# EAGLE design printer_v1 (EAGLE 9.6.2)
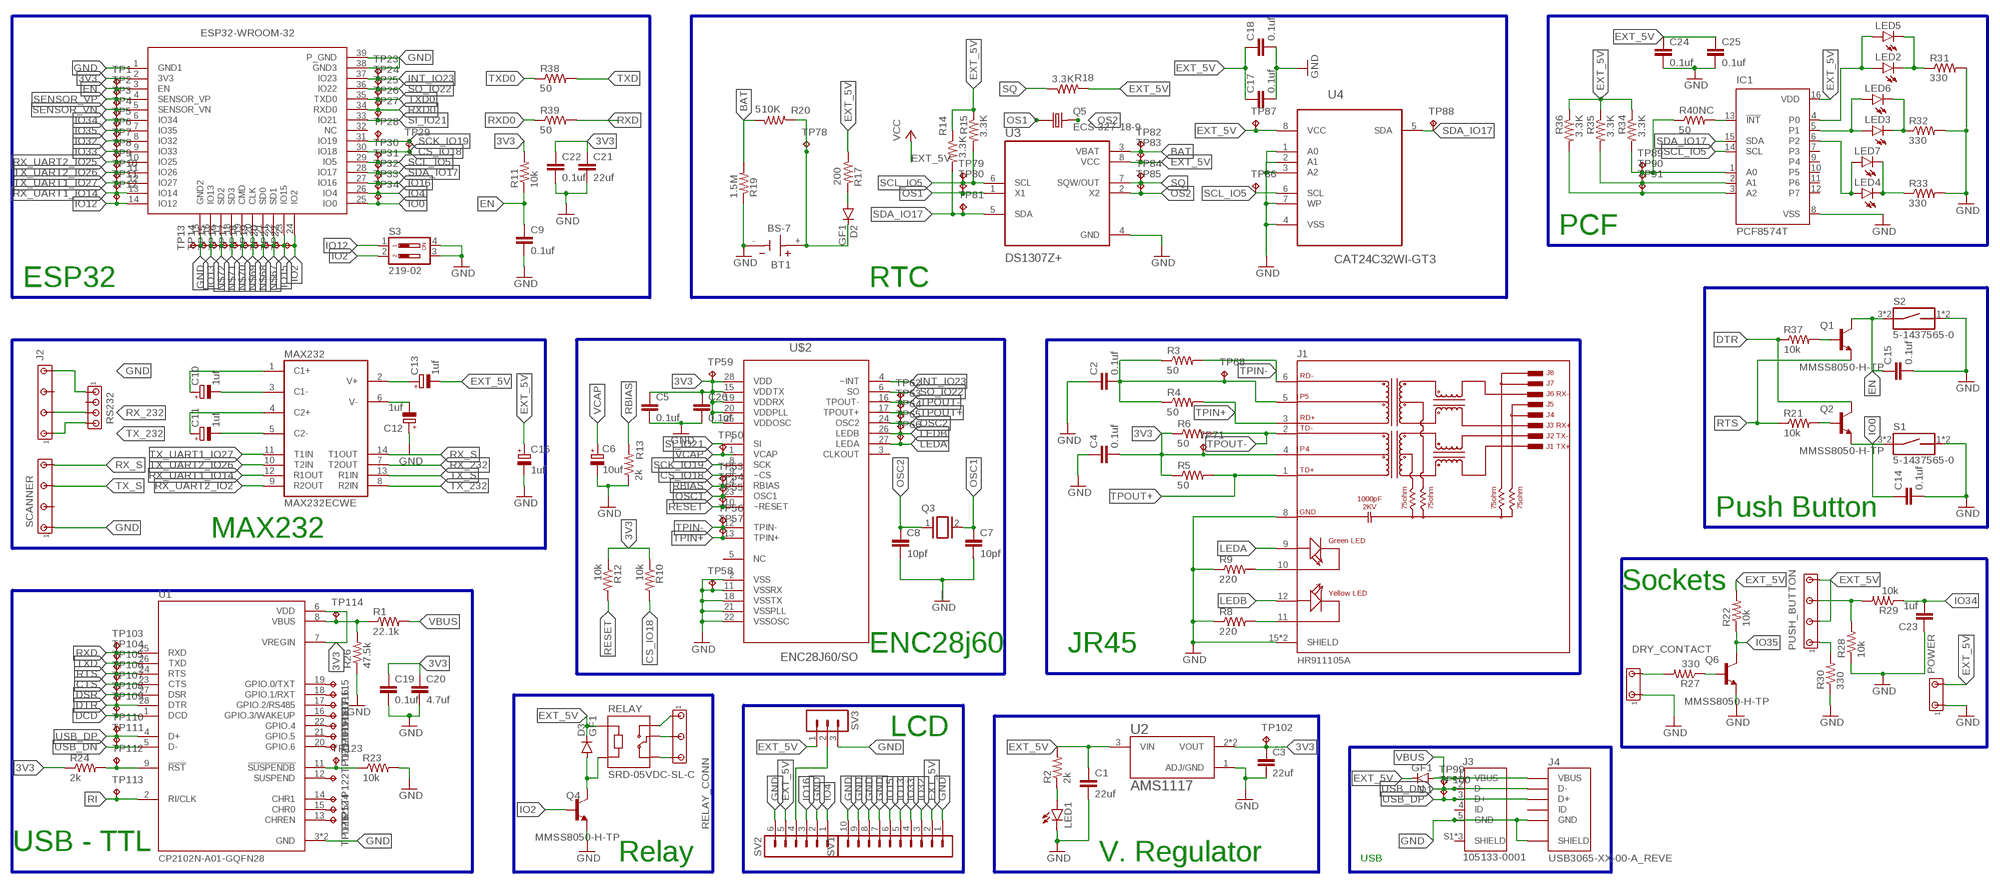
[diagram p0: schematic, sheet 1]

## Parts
BT1  BS-7  [BAT_BS-7]
C1  22uf  C-EUC1206  [C1206]
C2  0.1uf  C-EUC1206  [C1206]
C3  22uf  C-EUC1206  [C1206]
C4  0.1uf  C-EUC1206  [C1206]
C5  0.1uf  C-EUC1206  [C1206]
C6  10uf  CPOL-EU153CLV-0405  [153CLV-0405]
C7  10pf  C-EUC1206  [C1206]
C8  10pf  C-EUC1206  [C1206]
C9  0.1uf  C-EUC1206  [C1206]
C10  1uf  CPOL-EU153CLV-0405  [153CLV-0405]
C11  1uf  CPOL-EU153CLV-0405  [153CLV-0405]
C12  1uf  CPOL-EU153CLV-0405  [153CLV-0405]
C13  1uf  CPOL-EU153CLV-0405  [153CLV-0405]
C14  0.1uf  C-EUC1206  [C1206]
C15  0.1uf  C-EUC1206  [C1206]
C16  1uf  CPOL-EU153CLV-0405  [153CLV-0405]
C17  0.1uf  C-EUC1206  [C1206]
C18  0.1uf  C-EUC1206  [C1206]
C19  0.1uf  C-EUC1206  [C1206]
C20  4.7uf  C-EUC1206  [C1206]
C21  22uf  C-EUC1206  [C1206]
C22  0.1uf  C-EUC1206  [C1206]
C23  1uf  C-EUC1206  [C1206]
C24  0.1uf  C-EUC1206  [C1206]
C25  0.1uf  C-EUC1206  [C1206]
C26  0.1uf  C-EUC1206  [C1206]
D1  GF1  [SMA-DO214AC]
D2  GF1  [SMA-DO214AC]
D3  GF1  [SMA-DO214AC]
DRY_CONTACT  MTA03-100_MYV  [10X03MTA_MYV]
IC1  PCF8574T  [SO16W]
J1  HR911105A  [HANRUN_HR911105A]
J2  MTA07-100_MYV  [10X07MTA_MYV]
J3  105133-0001  [MOLEX_105133-0001]
J4  USB3065-XX-00-A_REVE  [GCT_USB3065-XX-00-A_REVE]
LED1  LEDSML0603  [SML0603]
LED2  LEDSML0603  [SML0603]
LED3  LEDSML0603  [SML0603]
LED4  LEDSML0603  [SML0603]
LED5  LED5MM  [LED5MM]
LED6  LED5MM  [LED5MM]
LED7  LED5MM  [LED5MM]
MAX232  MAX232ECWE  [SO16L]
POWER  MTA03-100_MYV  [10X03MTA_MYV]
PUSH_BUTTON  MTA07-100_MYV  [10X07MTA_MYV]
Q1  MMSS8050-H-TP  [TRANS_MMSS8050-H-TP]
Q2  MMSS8050-H-TP  [TRANS_MMSS8050-H-TP]
Q3  XTAL/S  [QS]
Q4  MMSS8050-H-TP  [TRANS_MMSS8050-H-TP]
Q5  ECS-327-18-9  [XTAL_ECS-160-18-9X]
Q6  MMSS8050-H-TP  [TRANS_MMSS8050-H-TP]
R1  22.1k  R-US_R1206  [R1206]
R2  2k  R-US_R1206  [R1206]
R3  50  R-US_R1206  [R1206]
R4  50  R-US_R1206  [R1206]
R5  50  R-US_R1206  [R1206]
R6  50  R-US_R1206  [R1206]
R8  220  R-US_R1206  [R1206]
R9  220  R-US_R1206  [R1206]
R10  10k  R-US_R0805  [R0805]
R11  10k  R-US_R0805  [R0805]
R12  10k  R-US_R0805  [R0805]
R13  2k  R-US_R1206  [R1206]
R14  3.3K  R-US_R1206  [R1206]
R15  3.3K  R-US_R1206  [R1206]
R17  200  R-US_R1206  [R1206]
R18  3.3K  R-US_R1206  [R1206]
R19  1.5M  R-US_R1206  [R1206]
R20  510K  R-US_R1206  [R1206]
R21  10k  R-US_R0805  [R0805]
R22  10k  R-US_R0805  [R0805]
R23  10k  R-US_R0805  [R0805]
R24  2k  R-US_R1206  [R1206]
R26  47.5k  R-US_R1206  [R1206]
R27  330  R-US_R0402  [R0402]
R28  10k  R-US_R0805  [R0805]
R29  10k  R-US_R0805  [R0805]
R30  330  R-US_R1206  [R1206]
R31  330  R-US_R1206  [R1206]
R32  330  R-US_R1206  [R1206]
R33  330  R-US_R1206  [R1206]
R34  3.3K  R-US_R1206  [R1206]
R35  3.3K  R-US_R1206  [R1206]
R36  3.3K  R-US_R1206  [R1206]
R37  10k  R-US_R0805  [R0805]
R38  50  R-US_R0402  [R0402]
R39  50  R-US_R0402  [R0402]
R40NC  50  R-US_R0402  [R0402]
RELAY  SRD-05VDC-SL-C  [RELAY_SRD-05VDC-SL-C]
RELAY_CONN  MTA05-156_MYVSPACE1  [10X05MTA_MYV]
RS232  MTA04-100  [10X04MTA]
S1  5-1437565-0  [SW_5-1437565-0]
S2  5-1437565-0  [SW_5-1437565-0]
S3  219-02  [CTS-219-02]
SCANNER  MTA07-100_MYV  [10X07MTA_MYV]
SV1  MA10-1  [MA10-1]
SV2  MA06-1  [MA06-1]
SV3  MA03-1  [MA03-1]
TP1  TPTP06R  [TP06R]
TP2  TPTP06R  [TP06R]
TP3  TPTP06R  [TP06R]
TP4  TPTP06R  [TP06R]
TP5  TPTP06R  [TP06R]
TP6  TPTP06R  [TP06R]
TP7  TPTP06R  [TP06R]
TP8  TPTP06R  [TP06R]
TP9  TPTP06R  [TP06R]
TP10  TPTP06R  [TP06R]
TP11  TPTP06R  [TP06R]
TP12  TPTP06R  [TP06R]
TP13  TPTP06R  [TP06R]
TP14  TPTP06R  [TP06R]
TP15  TPTP06R  [TP06R]
TP16  TPTP06R  [TP06R]
TP17  TPTP06R  [TP06R]
TP18  TPTP06R  [TP06R]
TP19  TPTP06R  [TP06R]
TP20  TPTP06R  [TP06R]
TP21  TPTP06R  [TP06R]
TP22  TPTP06R  [TP06R]
TP23  TPTP06R  [TP06R]
TP24  TPTP06R  [TP06R]
TP25  TPTP06R  [TP06R]
TP26  TPTP06R  [TP06R]
TP27  TPTP06R  [TP06R]
TP28  TPTP06R  [TP06R]
TP29  TPTP06R  [TP06R]
TP30  TPTP06R  [TP06R]
TP31  TPTP06R  [TP06R]
TP32  TPTP06R  [TP06R]
TP33  TPTP06R  [TP06R]
TP34  TPTP06R  [TP06R]
TP50  TPTP06R  [TP06R]
TP53  TPTP06R  [TP06R]
TP54  TPTP06R  [TP06R]
TP55  TPTP06R  [TP06R]
TP56  TPTP06R  [TP06R]
TP57  TPTP06R  [TP06R]
TP58  TPTP06R  [TP06R]
TP59  TPTP06R  [TP06R]
TP62  TPTP06R  [TP06R]
TP63  TPTP06R  [TP06R]
TP64  TPTP06R  [TP06R]
TP65  TPTP06R  [TP06R]
TP66  TPTP06R  [TP06R]
TP68  TPTP06R  [TP06R]
TP71  TPTP06R  [TP06R]
TP78  TPTP06R  [TP06R]
TP79  TPTP06R  [TP06R]
TP80  TPTP06R  [TP06R]
TP81  TPTP06R  [TP06R]
TP82  TPTP06R  [TP06R]
TP83  TPTP06R  [TP06R]
TP84  TPTP06R  [TP06R]
TP85  TPTP06R  [TP06R]
TP86  TPTP06R  [TP06R]
TP87  TPTP06R  [TP06R]
TP88  TPTP06R  [TP06R]
TP89  TPTP06R  [TP06R]
TP90  TPTP06R  [TP06R]
TP91  TPTP06R  [TP06R]
TP99  TPTP06R  [TP06R]
TP100  TPTP06R  [TP06R]
TP102  TPTP06R  [TP06R]
TP103  TPTP06R  [TP06R]
TP104  TPTP06R  [TP06R]
TP105  TPTP06R  [TP06R]
TP106  TPTP06R  [TP06R]
TP107  TPTP06R  [TP06R]
TP108  TPTP06R  [TP06R]
TP109  TPTP06R  [TP06R]
TP110  TPTP06R  [TP06R]
TP111  TPTP06R  [TP06R]
TP112  TPTP06R  [TP06R]
TP113  TPTP06R  [TP06R]
TP114  TPTP06R  [TP06R]
TP115  TPTP06R  [TP06R]
TP116  TPTP06R  [TP06R]
TP117  TPTP06R  [TP06R]
TP118  TPTP06R  [TP06R]
TP119  TPTP06R  [TP06R]
TP120  TPTP06R  [TP06R]
TP121  TPTP06R  [TP06R]
TP122  TPTP06R  [TP06R]
TP123  TPTP06R  [TP06R]
TP124  TPTP06R  [TP06R]
TP125  TPTP06R  [TP06R]
TP126  TPTP06R  [TP06R]
U1  CP2102N-A01-GQFN28  [QFN50P500X500X80-29N]
U2  AMS1117  [SOT229P700X180-4N]
U3  DS1307Z+  [SOIC127P600X175-8N]
U4  CAT24C32WI-GT3  [SOIC127P600X175-8N]
U$2  ENC28J60/SO  [SOIC127P1034X264-28N]
U$3  ESP32-WROOM-32  [ESP32-WROOM-32]

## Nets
3V3 [POWER]: C3.1 C4.2 C5.1 C19.1 C20.1 C21.1 C22.1 C26.1 J1.4 R5.1 R6.1 R10.1 R11.2 R12.1 R24.1 TP59.TP TP71.TP TP102.TP U1.6(VDD) U1.7(VREGIN) U2.2(VOUT) U2.4(VOUT) U$2.15(VDDTX) U$2.19(VDDRX) U$2.20(VDDPLL) U$2.25(VDDOSC) U$2.28(VDD) U$3.2(3V3)
BAT: R19.2 R20.2 TP82.TP U3.3(VBAT)
CS_IO18: R10.2 TP29.TP U$2.9(~CS) U$3.30(IO18)
CTS: TP106.TP U1.23(CTS)
DCD: TP109.TP U1.1(DCD)
DSR: TP107.TP U1.27(DSR)
DTR: Q2.3(C) R37.1 TP108.TP U1.28(DTR)
EN: C9.1 C15.1 Q1.3(C) R11.1 S2.3 S2.4 TP1.TP U$3.3(EN)
EXT_5V [POWER]: C1.1 C13.- C16.+ C17.1 C18.1 C24.1 C25.1 D1.K(C) D3.K(C) IC1.16(VDD) POWER.3 PUSH_BUTTON.3 PUSH_BUTTON.7 R2.2 R14.1 R15.1 R17.1 R18.2 R22.2 R34.1 R35.1 R36.1 RELAY.A1 SV1.2 SV2.5 SV3.1 TP83.TP TP87.TP U2.3(VIN) U3.8(VCC) U4.8(VCC) ; supply symbol labelled VCC
GND [POWER]: BT1.- C1.2 C2.1 C3.2 C4.1 C5.2 C6.- C7.2 C8.2 C9.2 C12.+ C14.2 C15.2 C16.- C17.2 C18.2 C19.2 C20.2 C21.2 C22.2 C23.1 C24.2 C25.2 C26.2 DRY_CONTACT.1 IC1.8(VSS) J1.8(GND) J1.15(SHIELD) J1.16(SHIELD) J2.7 J3.5(GND) J4.5(GND) J4.6(SHIELD) J4.7(SHIELD) J4.8(SHIELD) J4.9(SHIELD) LED1.C POWER.1 Q4.2(E) Q6.2(E) R8.1 R9.1 R13.1 R19.1 R23.2 R26.1 R28.1 R30.1 R31.2 R32.2 R33.2 RS232.1 S1.1 S1.2 S2.1 S2.2 S3.3 S3.4 SCANNER.1 SV1.1 SV1.7 SV1.8 SV1.9 SV1.10 SV2.2 SV2.6 SV3.3 TP13.TP TP58.TP U1.3(GND) U1.29(GND) U2.1(ADJ/GND) U3.4(GND) U4.1(A0) U4.2(A1) U4.3(A2) U4.4(VSS) U4.7(WP) U$2.2(VSS) U$2.11(VSSRX) U$2.18(VSSTX) U$2.21(VSSPLL) U$2.22(VSSOSC) U$3.1(GND1) U$3.15(GND2) U$3.38(GND3) U$3.39(P_GND)
INT_IO23: TP23.TP U$2.4(~INT) U$3.37(IO23)
IO0: C14.1 Q2.2(E) S1.3 S1.4 TP34.TP U$3.25(IO0)
IO2: Q4.1(B) S3.2 TP22.TP U$3.24(IO2)
IO4: SV2.1 TP33.TP U$3.26(IO4)
IO12: S3.1 TP12.TP U$3.14(IO12)
IO13: SV1.5 TP14.TP U$3.16(IO13)
IO15: SV1.6 TP21.TP U$3.23(IO15)
IO16: SV2.3 TP32.TP U$3.27(IO16)
IO32: SV1.3 TP6.TP U$3.8(IO32)
IO33: SV1.4 TP7.TP U$3.9(IO33)
IO34: C23.2 R29.1 TP4.TP U$3.6(IO34)
IO35: Q6.3(C) R22.1 TP5.TP U$3.7(IO35)
LEDA: J1.9(GA) TP66.TP U$2.27(LEDA)
LEDB: J1.12(YA) TP65.TP U$2.26(LEDB)
N$1: LED1.A R2.1
N$2: Q1.1(B) R37.2
N$3: Q2.1(B) R21.2
N$4: R1.1 R26.2 TP114.TP U1.8(VBUS)
N$5: SV2.4 SV3.2
N$6: R23.1 TP123.TP U1.11(!SUSPENDB)
N$7: J1.11(YC) R8.2
N$8: C2.2 J1.5 R3.1 R4.1 TP68.TP
N$9: J1.10(GC) R9.2
N$10: TP115.TP U1.19(GPIO.0/TXT)
N$11: TP116.TP U1.18(GPIO.1/RXT)
N$12: C10.+ MAX232.1(C1+)
N$13: TP117.TP U1.17(GPIO.2/RS485)
N$14: C10.- MAX232.3(C1-)
N$15: C11.- MAX232.5(C2-)
N$16: R24.2 TP112.TP U1.9(!RST)
N$17: TP118.TP U1.16(GPIO.3/WAKEUP)
N$18: C11.+ MAX232.4(C2+)
N$19: C12.- MAX232.6(V-)
N$20: C13.+ MAX232.2(V+)
N$21: RELAY.NC RELAY_CONN.5
N$22: RELAY.COM RELAY_CONN.3
N$23: LED2.C LED5.K(C) R31.1
N$24: IC1.13(!INT) R40NC.2
N$25: TP119.TP U1.22(GPIO.4)
N$26: RELAY.NO RELAY_CONN.1
N$27: D3.A Q4.3(C) RELAY.A2
N$28: D2.A R17.2
N$29: BT1.+ D2.K(C) R20.1 TP78.TP
N$30: TP120.TP U1.21(GPIO.5)
N$31: TP121.TP U1.20(GPIO.6)
N$32: Q6.1(B) R27.1
N$33: PUSH_BUTTON.5 R28.2 R29.2
N$34: TP122.TP U1.12(SUSPEND)
N$35: DRY_CONTACT.3 R27.2
N$36: IC1.4(P0) LED2.A LED5.A
N$37: IC1.5(P1) LED3.A LED6.A
N$38: IC1.6(P2) LED4.A LED7.A
N$39: TP124.TP U1.14(CHR1)
N$40: PUSH_BUTTON.1 R30.2
N$41: TP125.TP U1.15(CHR0)
N$42: TP126.TP U1.13(CHREN)
N$45: IC1.1(A0) R34.2 R40NC.1 TP89.TP
N$46: IC1.2(A1) R35.2 TP90.TP
N$47: IC1.3(A2) R36.2 TP91.TP
N$48: LED3.C LED6.K(C) R32.1
N$49: LED4.C LED7.K(C) R33.1
N$67: TP20.TP U$3.22(SD1)
N$68: TP19.TP U$3.21(SD0)
N$69: TP18.TP U$3.20(CLK)
N$70: TP17.TP U$3.19(CMD)
N$71: TP16.TP U$3.18(SD3)
N$72: TP15.TP U$3.17(SD2)
OS1: Q5.1 TP80.TP U3.1(X1)
OS2: Q5.2 TP85.TP U3.2(X2)
OSC1: C7.1 Q3.2 TP54.TP U$2.23(OSC1)
OSC2: C8.1 Q3.1 TP64.TP U$2.24(OSC2)
RBIAS: R13.2 TP53.TP U$2.14(RBIAS)
RESET: R12.2 TP55.TP U$2.10(~RESET)
RI: TP113.TP U1.2(RI/CLK)
RTS: Q1.2(E) R21.1 TP105.TP U1.24(RTS)
RX_232: J2.3 MAX232.7(T2OUT) RS232.3
RX_S: MAX232.14(T1OUT) SCANNER.7
RX_UART1_IO14: MAX232.12(R1OUT) TP11.TP U$3.13(IO14)
RX_UART2_IO2: MAX232.9(R2OUT)
RX_UART2_IO25: TP8.TP U$3.10(IO25)
RXD: R39.2 TP103.TP U1.25(RXD)
RXD0: R39.1 TP26.TP U$3.34(RXD0)
SCK_IO19: TP28.TP U$2.8(SCK) U$3.31(IO19)
SCL_IO5: IC1.14(SCL) R15.2 TP30.TP TP79.TP TP86.TP U3.6(SCL) U4.6(SCL) U$3.29(IO5)
SDA_IO17: IC1.15(SDA) R14.2 TP31.TP TP81.TP TP88.TP U3.5(SDA) U4.5(SDA) U$3.28(IO17)
SENSOR_VN: TP3.TP U$3.5(SENSOR_VN)
SENSOR_VP: TP2.TP U$3.4(SENSOR_VP)
SI_IO21: TP27.TP U$2.7(SI) U$3.33(IO21)
SO_IO22: TP24.TP U$2.6(SO) U$3.36(IO22)
SQ: R18.1 TP84.TP U3.7(SQW/OUT)
TPIN+: J1.3(RD+) R4.2 TP57.TP U$2.13(TPIN+)
TPIN-: J1.6(RD-) R3.2 TP56.TP U$2.12(TPIN-)
TPOUT+: J1.1(TD+) R5.2 TP63.TP U$2.17(TPOUT+)
TPOUT-: J1.2(TD-) R6.2 TP62.TP U$2.16(TPOUT-)
TX_232: J2.1 MAX232.8(R2IN) RS232.4
TX_S: MAX232.13(R1IN) SCANNER.5
TX_UART1_IO27: MAX232.11(T1IN) TP10.TP U$3.12(IO27)
TX_UART2_IO26: MAX232.10(T2IN) TP9.TP U$3.11(IO26)
TXD: R38.2 TP104.TP U1.26(TXD)
TXD0: R38.1 TP25.TP U$3.35(TXD0)
USB_DN: J3.2(D-) J4.2(D-) TP99.TP TP111.TP U1.5(D-)
USB_DP: J3.3(D+) J4.3(D+) TP100.TP TP110.TP U1.4(D+)
VBUS [POWER]: D1.A J3.1(VBUS) J4.1(VBUS) R1.2
VCAP: C6.+ TP50.TP U$2.1(VCAP)
Unconnected: IC1.7(P3) IC1.9(P4) IC1.10(P5) IC1.11(P6) IC1.12(P7) J2.5 J3.4(ID) J3.S1(SHIELD) J3.S2(SHIELD) J3.S3(SHIELD) J4.4(ID) RS232.2 SCANNER.3 U$2.3(CLKOUT) U$2.5(NC) U$3.32(NC)

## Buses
B$1
B$2
BAT,EXT_5V,GND,N$28,N$29
B$3
B$4
B$5
B$6
B$7
GND,EXT_5V_PIN
B$8
VBUS,GND,USB_DN,N$6,3V3,RI,RTS,RXD,TXD,CTS,DSR,N$4,DTR,DCD,USB_DP,N$16
B$9
B$10

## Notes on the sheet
- PCF
- ESP32 | RTC
- Push Button
- MAX232
- Sockets
- ENC28j60 | JR45
- LCD
- USB - TTL
- Relay | V. Regulator | USB

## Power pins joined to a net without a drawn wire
EXT_5V: MAX232.16(VCC)
GND: MAX232.15(GND)

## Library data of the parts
BT1 = BS-7:BS-7: BATTERY HOLDER COIN 20MM PC PIN; AVAILABILITY: Unavailable; DESCRIPTION: BATTERY HOLDER COIN 20MM PC PIN; MF: MPD _Memory; MP: BS-7; PACKAGE: None; PRICE: None
C1-C5 C7-C9 C14 C15 C17-C26 = rcl:C-EU: CAPACITOR, European symbol; SPICEPREFIX: C
C6 C10-C13 C16 = rcl:CPOL-EU: POLARIZED CAPACITOR, European symbol; SPICEPREFIX: C
D1-D3 = diode:GF1: DIODE
DRY_CONTACT POWER = con-amp_edit:MTA03-100_MYV: AMP connector
IC1 = micro-philips:PCF8574: I2C-Bus Remote 8-bit I/O expander http://www.semiconductors.philips.com/acrobat_download/datasheets/PCF8574_4.pdf; MPN: PCF8574T/3,512; OC_FARNELL: 1201255; OC_NEWARK: 70R6870
J1 = HR911105A:HR911105A: DIP RJ45 Connector;; AVAILABILITY: Unavailable; DESCRIPTION: HR911105A Ethernet Interface Arduino Platform Evaluation Expansion Board; MF: DFRobot; MP: HR911105A; PACKAGE: None; PRICE: None
J2 PUSH_BUTTON SCANNER = con-amp_edit:MTA07-100_MYV: AMP connector
J3 = 105133-0001:105133-0001: Conn Micro USB Type B RCP 5 POS 0.65mm Solder RA SMD 5 Terminal 1 Port Embossed T/R; AVAILABILITY: Unavailable; DESCRIPTION: USB - micro B USB 2.0 Receptacle Connector 5 Position Surface Mount; MF: Molex; MP: 105133-0001; PACKAGE: None; PRICE: None
J4 = USB3065-XX-00-A_REVE:USB3065-XX-00-A_REVE: Micro USB Receptacle, Type B, 5 Pin, SMT, Horizontal, Bottom Mount (Standart), Optional Plastic Locating Peg; AVAILABILITY: Unavailable; DESCRIPTION: USB3065 Series 5 Pin, SMT, Horizontal, Bottom Mount, Micro USB Receptacle; MF: Global Connector Technology; MP: USB3065-30-00-A; PACKAGE: None; PRICE: None
LED1-LED4 = led:LED: LED
LED5-LED7 = led_MYVV:LED: LED
MAX232 = maxim:MAX232ECWE: RS232 TRANSCEIVER; MF: MAXIM; MPN: MAX232ECWE+; OC_FARNELL: 9724435; OC_NEWARK: 67K4440
Q1 Q2 Q4 Q6 = MMSS8050-H-TP:MMSS8050-H-TP: MMSS8050-H Series 25 V 1.5 A NPN Silicon Plastic-Encapsulate Transistor-SOT-23; AVAILABILITY: Unavailable; DESCRIPTION: Bipolar _BJT_ Transistor NPN 25V 1.5A 100MHz 625mW Surface Mount SOT-23; MF: Micro Commercial; MP: MMSS8050-H-TP; PACKAGE: SOT-23 Micro Commercial; PRICE: None
Q3 = special:XTAL/S: CRYSTAL
Q5 = ECS-327-18-9:ECS-327-18-9: Crystal Cylindrical Can, Radial; AVAILABILITY: Unavailable; DESCRIPTION: 32.768MHz ±50ppm Crystal 18pF 100 Ohms Cylindrical Can, Radial; MF: ECS International; MP: ECS-327-18-9; PACKAGE: Cylindrical Can Radial ECS International; PRICE: None
R1-R6 R8-R15 R17-R24 R26-R39 R40NC = rcl:R-US_: RESISTOR, American symbol; SPICEPREFIX: R
RELAY = SRD-05VDC-SL-C:SRD-05VDC-SL-C: 5V Trigger Relay Module For Arduino And Raspberry Pi 5V Trigger Relay Module For Arduino And Raspberry Pi; AVAILABILITY: Unavailable; DESCRIPTION: 5V Trigger Relay Module For Arduino And Raspberry Pi 5V Trigger Relay Module For Arduino And Raspberry Pi; MF: Songle Relay; MP: SRD-05VDC-SL-C; PACKAGE: None; PRICE: None
RELAY_CONN = con-amp_edit:MTA05-156_MYV: AMP connector
RS232 = con-amp:MTA04-100: AMP connector
S1 S2 = 5-1437565-0:5-1437565-0: Switch Tactile OFF (ON) Round Button Gull Wing 0.05A 12VDC 1.57N SMD T/R; AVAILABILITY: Unavailable; COMMENT: 5-1437565-0; DESCRIPTION: Switch Push Button N.O. SPST Round Button 0.05A 12VDC 1VA Alternate Contact Gull Wing SMD T/R; MF: TE Connectivity; MP: FSM6JSMATR; PACKAGE: None; PRICE: None; TE_PURCHASE_URL: https://www.te.com/usa-en/product-5-1437565-0.html?te_bu=Cor&te_type=disp&te_campaign=seda_glo_cor-seda-global-disp-prtnr-fy19-seda-model-bom-cta_sma-317_1&elqCampaignId=32493
S3 = switch-dil:219-02*: Surface Mount DIP Switch Series 219 SMT CTS Electronic Components Sourc: www.ctscorp.com; OC_FARNELL: unknown; OC_NEWARK: unknown
SV1 = con-lstb:MA10-1: PIN HEADER; OC_FARNELL: unknown; OC_NEWARK: unknown
SV2 = con-lstb:MA06-1: PIN HEADER; OC_FARNELL: unknown; OC_NEWARK: unknown
SV3 = con-lstb:MA03-1: PIN HEADER; OC_FARNELL: unknown; OC_NEWARK: unknown
TP1-TP34 TP50 TP53-TP59 TP62-TP66 TP68 TP71 TP78-TP91 TP99 TP100 TP102-TP126 = testpad:TP: Test pad
U1 = CP2102N-A01-GQFN28:CP2102N-A01-GQFN28: Ic Bridge Usb To Uart 28qfn; DESCRIPTION: USB Bridge, USB to UART USB 2.0 UART Interface 28-QFN _5x5_; DIGI-KEY_PART_NUMBER: 336-3694-ND; DIGI-KEY_PURCHASE_URL: https://www.digikey.com/product-detail/en/silicon-labs/CP2102N-A01-GQFN28/336-3694-ND/6012519?utm_source=snapeda&utm_medium=aggregator&utm_campaign=symbol; MF: Silicon Labs; MP: CP2102N-A01-GQFN28; PACKAGE: QFN-28 Silicon Labs
U2 = AMS1117:AMS1117: Sot223/Pkg 1-Amp 5-Volt Low Drop Out Voltage Regulatator; AVAILABILITY: Unavailable; DESCRIPTION: UNO PLUS Arduino R3 Shield, Xbee Arduino IDE Wheeled Robotics Kit; MF: Seeed Technology; MP: AMS1117; PACKAGE: SOT-223 Seeed Technology; PRICE: None
U3 = DS1307Z_:DS1307Z+; AVAILABILITY: Unavailable; DESCRIPTION: Real Time Clock _RTC_ IC Clock/Calendar 56B I²C, 2-Wire Serial 8-SOIC _0.154, 3.90mm Width_; MF: Maxim Integrated; MP: DS1307Z; PACKAGE: SO-8 Maxim Integrated; PRICE: None
U4 = CAT24C32WI-GT3:CAT24C32WI-GT3: 32-Kb I2C CMOS Serial EEPROM; AVAILABILITY: Unavailable; DESCRIPTION: EEPROM Memory IC 32Kb _4K x 8_ I²C 1MHz 400ns 8-SOIC; MF: ON; MP: CAT24C32WI-GT3; PACKAGE: SOIC-8 ON; PRICE: None
U$2 = ENC28J60_SO:ENC28J60/SO: Stand-Alone Ethernet Controller;; AVAILABILITY: Unavailable; DESCRIPTION: Ethernet Controller 10 Base-T PHY SPI Interface 28-SSOP; MF: Microchip; MP: ENC28J60/SS; PACKAGE: SSOP-28 Microchip; PRICE: None
U$3 = ESP32-WROOM-32:ESP32-WROOM-32: ESP32-WROOM-32 Module; AVAILABILITY: Unavailable; DESCRIPTION: Bluetooth, WiFi Transceiver Module 2.4GHz ~ 2.5GHz Surface Mount; MF: Espressif Systems; MP: ESP32-WROOM-32; PACKAGE: Module Espressif Systems; PRICE: None

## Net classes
1 POWER: width 0.254 mm

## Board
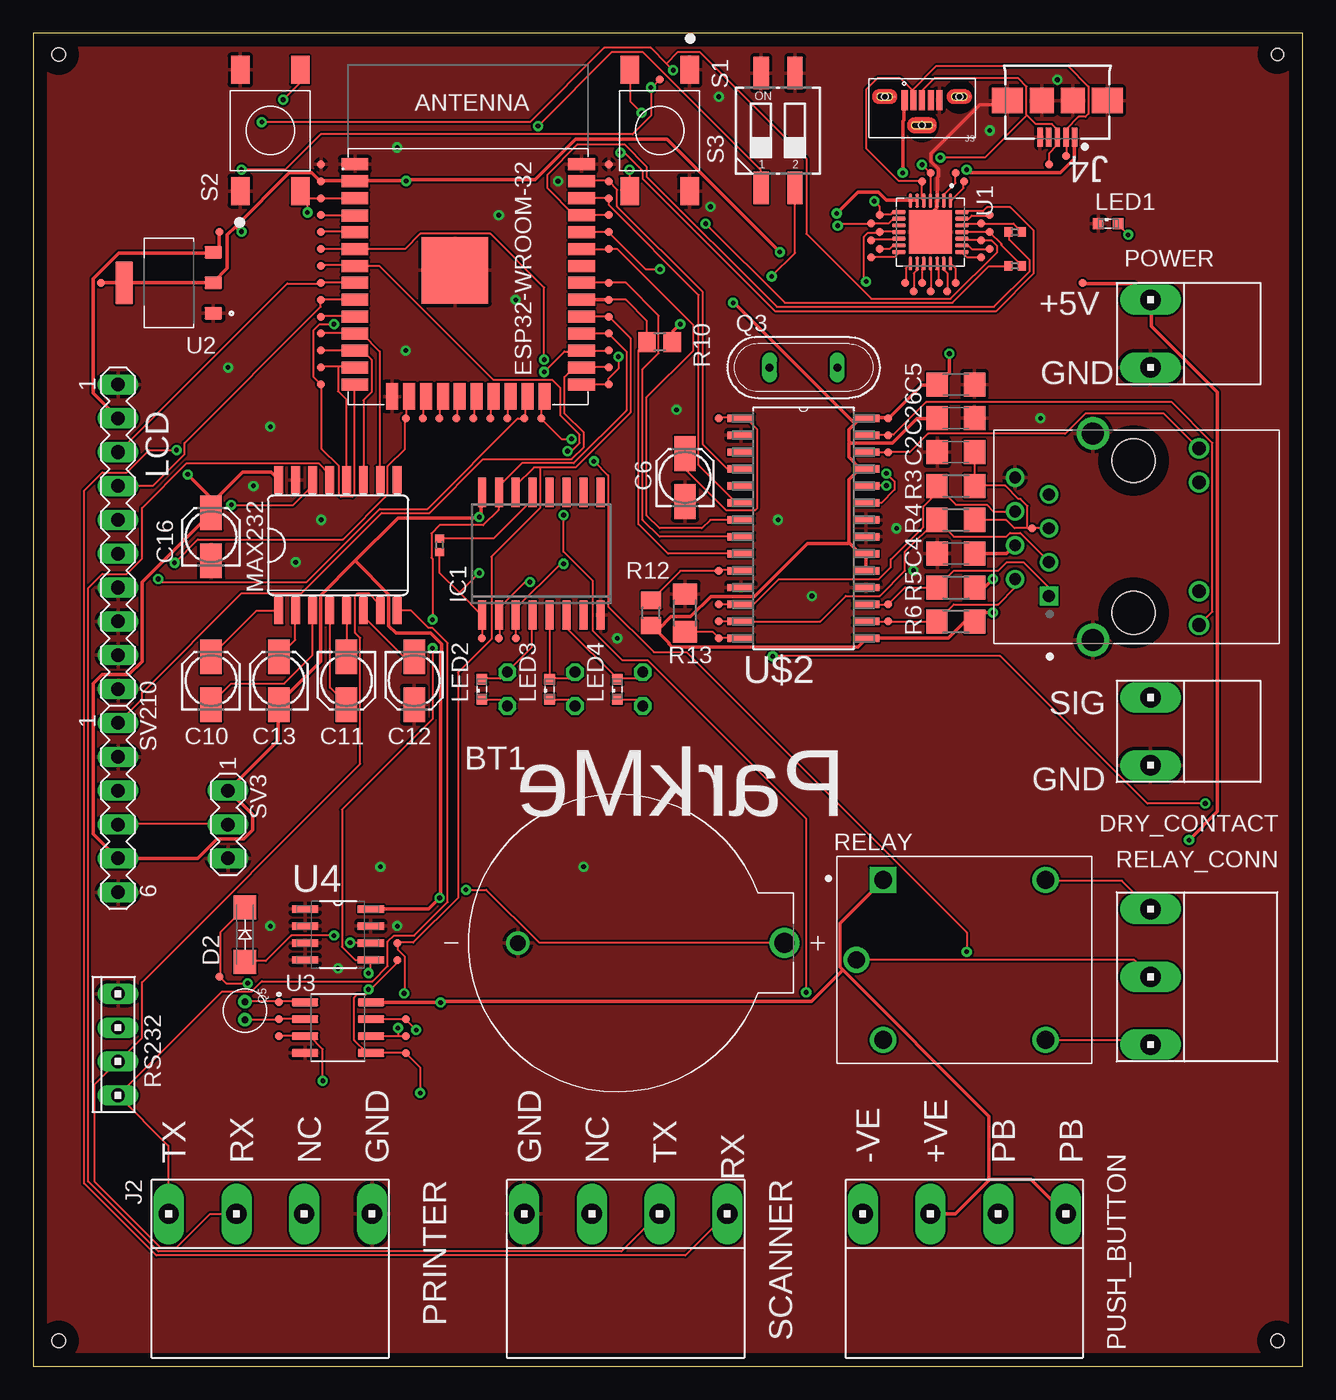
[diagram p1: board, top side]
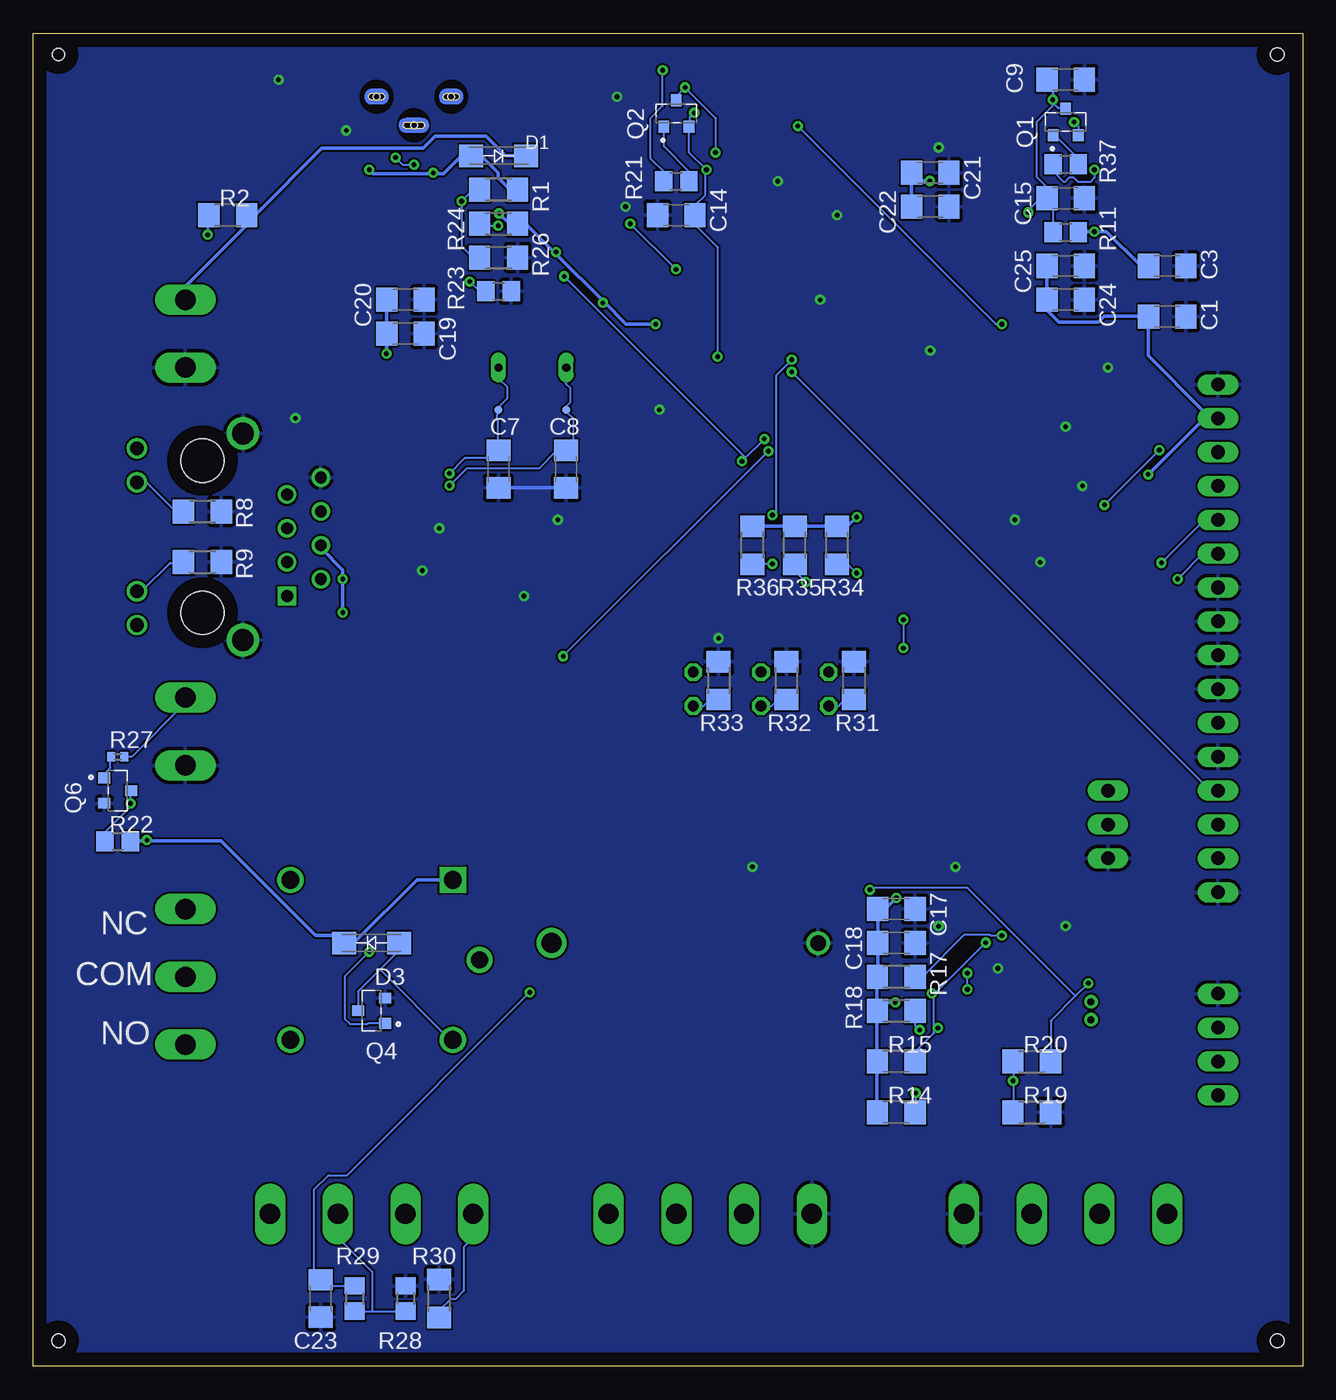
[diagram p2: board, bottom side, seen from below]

Size 95.23 x 100 mm. Coordinates in mm from the lower left corner, seen from the top.
Outline: 0,0 95.23,0 95.23,100 0,100 0,0
Copper layers (1*16): Top 0.035mm / dielectric 1.5mm / Bottom 0.035mm
Design rules "default": minimum track width 6mil, minimum drill 0.35mm, track to track 6mil, track to pad 6mil, pad to pad 6mil, via to via 6mil, smd to smd 6mil, copper to edge 40mil, drill to drill 6mil, minimum pad ring 10mil, minimum via ring 8mil, stop-mask expansion 4mil, vias tented up to drill 0mil, thermal gap 10mil
Holes 1 mm at 1.91,1.91 93.34,1.91 1.91,98.42
Holes 0.9 mm at 93.34,98.42

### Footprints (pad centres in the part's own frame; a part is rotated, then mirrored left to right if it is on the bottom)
BAT_BS-7 = drill 1.5: + 10,0 | drill 1.17: - -10,0
C1206 = smd 1.6 x 1.8: 1 -1.4,0; 2 1.4,0
153CLV-0405 = smd 2.6 x 1.6: + 1.8,0; - -1.8,0
SMA-DO214AC = smd 1.8 x 1.7: A -2.05,0; K 2.05,0
10X03MTA_MYV = drill 1.524 long: 1 2.54,0; 3 -2.54,0
SO16W = smd 0.6 x 2.2: 1 -4.445,-4.6; 2 -3.175,-4.6; 3 -1.905,-4.6; 4 -0.635,-4.6; 5 0.635,-4.6; 6 1.905,-4.6; 7 3.175,-4.6; 8 4.445,-4.6; 9 4.445,4.6; 10 3.175,4.6; 11 1.905,4.6; 12 0.635,4.6; 13 -0.635,4.6; 14 -1.905,4.6; 15 -3.175,4.6; 16 -4.445,4.6
HANRUN_HR911105A = drill 0.89 square: 1 4.45,-6.35 | drill 0.89: 2 3.18,-8.89; 3 1.91,-6.35; 4 0.64,-8.89; 5 -0.63,-6.35; 6 -1.9,-8.89; 7 -3.17,-6.35; 8 -4.44,-8.89 | drill 1.02: 9 6.625,4.9; 10 4.085,4.9; 11 -4.085,4.9; 12 -6.625,4.9 | drill 1.63: 15 7.745,-3.05; 16 -7.745,-3.05 | hole 3.25: -5.715,0; 5.715,0
10X07MTA_MYV = drill 1.524 long: 1 7.62,0; 3 2.54,0; 5 -2.54,0; 7 -7.62,0
MOLEX_105133-0001 = smd 0.45 x 1.5: 1 -1.3,-0.25; 2 -0.65,-0.25; 3 0,-0.25; 4 0.65,-0.25; 5 1.3,-0.25 | smd 0.1 x 0.1: S1 -2.05,0; S2 3.55,0; S3 0.95,-2.15 | hole 0.5: -2.8,0; 2.8,0; 0,-2.15
GCT_USB3065-XX-00-A_REVE = smd 0.4 x 1.4: 1 -1.3,0.5; 2 -0.65,0.5; 3 0,0.5; 4 0.65,0.5; 5 1.3,0.5 | smd 1.8 x 1.9: 6 1.15,-2.25; 7 -1.15,-2.25 | smd 2.3 x 1.9: 8 3.75,-2.25; 9 -3.75,-2.25
SML0603 = smd 0.8 x 0.8: A 0.75,0; C -0.75,0
LED5MM = drill 0.813 octagon: A -1.27,0; K 1.27,0
SO16L = smd 0.66 x 2.032: 1 -4.445,-4.902; 2 -3.175,-4.902; 3 -1.905,-4.902; 4 -0.635,-4.902; 5 0.635,-4.902; 6 1.905,-4.902; 7 3.175,-4.902; 8 4.445,-4.902; 9 4.445,4.902; 10 3.175,4.902; 11 1.905,4.902; 12 0.635,4.902; 13 -0.635,4.902; 14 -1.905,4.902; 15 -3.175,4.902; 16 -4.445,4.902
TRANS_MMSS8050-H-TP = smd 0.9 x 0.8: 1 -1,0.95; 2 -1,-0.95; 3 1,0
QS = drill 0.61 long: 1 -2.54,0; 2 2.54,0
XTAL_ECS-160-18-9X = drill 0.52 pad 0.92: 1 -0.677,0; 2 0.677,0
R1206 = smd 1.6 x 1.803: 1 -1.422,0; 2 1.422,0
R0805 = smd 1.3 x 1.5: 1 -0.95,0; 2 0.95,0
R0402 = smd 0.6 x 0.7: 1 -0.5,0; 2 0.5,0
RELAY_SRD-05VDC-SL-C = drill 1.32 square: A1 -6.1,6 | drill 1.32: A2 -6.1,-6; NC 6.1,6; NO 6.1,-6 | drill 1.29: COM -8.1,0
10X05MTA_MYV = drill 1.524 long: 1 5.08,0; 3 0,0; 5 -5.08,0
10X04MTA = drill 1.016 long: 1 3.81,0; 2 1.27,0; 3 -1.27,0; 4 -3.81,0
SW_5-1437565-0 = smd 2.1 x 1.4: 1 -4.55,2.25; 2 4.55,2.25; 3 -4.55,-2.25; 4 4.55,-2.25
CTS-219-02 = smd 1.13 x 2.44: 1 -1.27,-4.3; 2 1.27,-4.3; 3 1.27,4.3; 4 -1.27,4.3
MA10-1 = drill 1.016 long: 1 -11.43,0; 2 -8.89,0; 3 -6.35,0; 4 -3.81,0; 5 -1.27,0; 6 1.27,0; 7 3.81,0; 8 6.35,0; 9 8.89,0; 10 11.43,0
MA06-1 = drill 1.016 long: 1 -6.35,0; 2 -3.81,0; 3 -1.27,0; 4 1.27,0; 5 3.81,0; 6 6.35,0
MA03-1 = drill 1.016 long: 1 -2.54,0; 2 0,0; 3 2.54,0
TP06R = smd 0.6 x 0.6: TP 0,0
QFN50P500X500X80-29N = smd 1.01 x 0.27: 1 -2.36,1.5; 2 -2.36,1; 3 -2.36,0.5; 4 -2.36,0; 5 -2.36,-0.5; 6 -2.36,-1; 7 -2.36,-1.5; 15 2.36,-1.5; 16 2.36,-1; 17 2.36,-0.5; 18 2.36,0; 19 2.36,0.5; 20 2.36,1; 21 2.36,1.5 | smd 0.27 x 1.01: 8 -1.5,-2.36; 9 -1,-2.36; 10 -0.5,-2.36; 11 0,-2.36; 12 0.5,-2.36; 13 1,-2.36; 14 1.5,-2.36; 22 1.5,2.36; 23 1,2.36; 24 0.5,2.36; 25 0,2.36; 26 -0.5,2.36; 27 -1,2.36; 28 -1.5,2.36 | smd 3.25 x 3.25: 29 0,0
SOT229P700X180-4N = smd 1.31 x 0.93: 1 -3.345,2.29; 2 -3.345,0; 3 -3.345,-2.29 | smd 1.31 x 3.24: 4 3.345,0
SOIC127P600X175-8N = smd 1.97 x 0.59: 1 -2.475,1.905; 2 -2.475,0.635; 3 -2.475,-0.635; 4 -2.475,-1.905; 5 2.475,-1.905; 6 2.475,-0.635; 7 2.475,0.635; 8 2.475,1.905
SOIC127P600X175-8N' = smd 1.981 x 0.559: 1 -2.464,1.905; 2 -2.464,0.635; 3 -2.464,-0.635; 4 -2.464,-1.905; 5 2.464,-1.905; 6 2.464,-0.635; 7 2.464,0.635; 8 2.464,1.905
SOIC127P1034X264-28N = smd 1.981 x 0.559: 1 -4.699,8.255; 2 -4.699,6.985; 3 -4.699,5.715; 4 -4.699,4.445; 5 -4.699,3.175; 6 -4.699,1.905; 7 -4.699,0.635; 8 -4.699,-0.635; 9 -4.699,-1.905; 10 -4.699,-3.175; 11 -4.699,-4.445; 12 -4.699,-5.715; 13 -4.699,-6.985; 14 -4.699,-8.255; 15 4.699,-8.255; 16 4.699,-6.985; 17 4.699,-5.715; 18 4.699,-4.445; 19 4.699,-3.175; 20 4.699,-1.905; 21 4.699,-0.635; 22 4.699,0.635; 23 4.699,1.905; 24 4.699,3.175; 25 4.699,4.445; 26 4.699,5.715; 27 4.699,6.985; 28 4.699,8.255
ESP32-WROOM-32 = smd 2 x 0.9: 1 0,0; 2 0,-1.27; 3 -0.01,-2.54; 4 0,-3.84; 5 0,-5.08; 6 0,-6.35; 7 0,-7.62; 8 0,-8.89; 9 0,-10.16; 10 0,-11.43; 11 0,-12.7; 12 0,-13.97; 13 0,-15.24; 14 0,-16.51; 25 16.999,-16.511; 26 16.999,-15.239; 27 17.001,-13.971; 28 16.999,-12.702; 29 16.997,-11.432; 30 16.999,-10.161; 31 17.002,-8.891; 32 17,-7.622; 33 17,-6.35; 34 17,-5.08; 35 17,-3.81; 36 17,-2.54; 37 17,-1.27; 38 17,0 | smd 0.9 x 2: 15 2.785,-17.41; 16 4.055,-17.41; 17 5.325,-17.41; 18 6.595,-17.41; 19 7.865,-17.41; 20 9.135,-17.41; 21 10.405,-17.41; 22 11.675,-17.41; 23 12.945,-17.41; 24 14.215,-17.41 | smd 5 x 5: 39 7.502,-7.946

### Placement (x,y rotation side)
BT1  46.35,31.75 0 top
C1  10.16,78.74 0 bottom
C2  69.22,68.58 0 top
C3  10.16,82.55 0 bottom
C4  69.22,60.96 0 top
C5  69.22,73.66 0 top
C6  48.9,66.67 90 top
C7  60.33,67.31 270 bottom
C8  55.24,67.31 270 bottom
C9  17.78,96.52 0 bottom
C10  13.34,51.44 90 top
C11  23.5,51.44 270 top
C12  28.57,51.44 270 top
C13  18.41,51.44 90 top
C14  46.99,86.36 180 bottom
C15  17.78,87.63 0 bottom
C16  13.34,62.23 90 top
C17  30.48,34.29 0 bottom
C18  30.48,31.75 0 bottom
C19  67.31,77.47 0 bottom
C20  67.31,80.01 0 bottom
C21  27.94,89.53 0 bottom
C22  27.94,87 0 bottom
C23  73.66,5.08 90 bottom
C24  17.78,80.01 0 bottom
C25  17.78,82.55 0 bottom
C26  69.22,71.12 0 top
D1  60.33,90.81 0 bottom
D2  15.88,32.38 90 top
D3  69.85,31.75 180 bottom
DRY_CONTACT  83.82,47.62 270 top
IC1  38.1,60.96 0 top
J1  82.55,62.23 270 top
J2  17.78,11.43 180 top
J3  66.67,95.25 0 top
J4  76.83,92.71 180 top
LED1  80.64,85.72 0 top
LED2  33.66,50.8 90 top
LED3  38.73,50.8 90 top
LED4  43.81,50.8 90 top
LED5  35.56,50.8 270 top
LED6  40.64,50.8 270 top
LED7  45.72,50.8 270 bottom
MAX232  22.86,61.59 0 top
POWER  83.82,77.47 270 top
PUSH_BUTTON  69.85,11.43 180 top
Q1  17.78,93.34 90 bottom
Q2  46.99,93.98 90 bottom
Q3  57.78,74.93 0 top
Q4  69.85,26.67 180 bottom
Q5  15.88,26.67 270 top
Q6  88.9,43.18 0 bottom
R1  60.33,88.27 0 bottom
R2  80.64,86.36 0 bottom
R3  69.22,66.04 180 top
R4  69.22,63.5 180 top
R5  69.22,58.42 180 top
R6  69.22,55.88 180 top
R8  82.55,64.14 180 bottom
R9  82.55,60.33 180 bottom
R10  46.99,76.83 180 top
R11  17.78,85.09 0 bottom
R12  46.35,56.52 90 top
R13  48.9,56.52 270 top
R14  30.48,19.05 0 bottom
R15  30.48,22.86 0 bottom
R17  30.48,29.21 0 bottom
R18  30.48,26.67 180 bottom
R19  20.32,19.05 180 bottom
R20  20.32,22.86 180 bottom
R21  46.99,88.9 0 bottom
R22  88.9,39.37 0 bottom
R23  60.33,80.64 0 bottom
R24  60.33,85.72 180 bottom
R26  60.33,83.19 180 bottom
R27  88.9,45.72 0 bottom
R28  67.31,5.08 270 bottom
R29  71.12,5.08 270 bottom
R30  64.77,5.08 270 bottom
R31  33.66,51.44 90 bottom
R32  38.73,51.44 90 bottom
R33  43.81,51.44 90 bottom
R34  34.92,61.59 270 bottom
R35  38.1,61.59 270 bottom
R36  41.27,61.59 270 bottom
R37  17.78,90.17 0 bottom
R38  73.66,85.09 0 top
R39  73.66,82.55 0 top
R40NC  30.48,61.59 90 top
RELAY  69.85,30.48 0 top
RELAY_CONN  83.82,29.21 270 top
RS232  6.35,24.13 90 top
S1  46.99,92.71 270 top
S2  17.78,92.71 90 top
S3  55.88,92.71 0 top
SCANNER  44.45,11.43 180 top
SV1  6.35,62.23 270 top
SV2  6.35,41.91 270 top
SV3  14.61,40.64 270 top
TP1  21.59,87.63 0 top
TP2  21.59,86.36 0 top
TP3  21.59,85.09 0 top
TP4  21.59,83.82 0 top
TP5  21.59,82.55 0 top
TP6  21.59,81.28 0 top
TP7  21.59,80.01 0 top
TP8  21.59,78.74 0 top
TP9  21.59,77.47 0 top
TP10  21.59,76.2 0 top
TP11  21.59,74.93 0 top
TP12  21.59,73.66 0 top
TP13  21.59,90.17 0 top
TP14  27.94,71.12 0 top
TP15  29.21,71.12 0 top
TP16  30.48,71.12 0 top
TP17  31.75,71.12 0 top
TP18  33.02,71.12 0 top
TP19  34.29,71.12 0 top
TP20  35.56,71.12 0 top
TP21  36.83,71.12 0 top
TP22  38.1,71.12 0 top
TP23  43.18,88.9 0 top
TP24  43.18,87.63 0 top
TP25  43.18,86.36 0 top
TP26  43.18,85.09 0 top
TP27  43.18,83.82 0 top
TP28  43.18,81.28 0 top
TP29  43.18,80.01 0 top
TP30  27.94,24.77 0 top
TP31  27.94,23.5 0 top
TP32  43.18,76.2 0 top
TP33  43.18,74.93 0 top
TP34  43.18,73.66 0 top
TP50  51.44,71.12 0 top
TP53  51.44,54.61 0 top
TP54  60.33,71.75 0 bottom
TP55  51.44,59.69 0 top
TP56  51.44,57.15 0 top
TP57  51.44,55.88 0 top
TP58  43.18,90.17 0 top
TP59  21.59,88.9 0 top
TP62  64.14,55.88 0 top
TP63  64.14,57.15 0 top
TP64  55.24,71.75 0 bottom
TP65  64.14,68.58 0 top
TP66  64.14,69.85 0 top
TP68  74.93,62.87 0 top
TP71  5.08,81.28 0 top
TP78  13.97,29.21 0 top
TP79  27.3,31.75 0 top
TP80  18.41,27.3 0 top
TP81  27.3,30.48 0 top
TP82  18.41,24.77 0 top
TP83  13.97,85.09 90 top
TP84  27.94,26.04 0 top
TP85  18.41,26.04 0 top
TP86  43.18,78.74 0 top
TP87  78.74,81.28 0 top
TP88  43.18,77.47 0 top
TP89  33.66,54.61 0 top
TP90  34.92,54.61 0 top
TP91  36.2,54.61 0 top
TP99  66.67,88.9 0 top
TP100  67.31,89.53 0 top
TP102  64.14,71.12 0 top
TP103  71.75,85.09 0 top
TP104  71.12,85.72 0 top
TP105  71.12,84.45 0 top
TP106  71.75,83.82 0 top
TP107  71.75,86.36 0 top
TP108  46.99,96.52 0 top
TP109  69.85,88.9 0 top
TP110  76.2,90.17 0 top
TP111  77.47,90.81 0 top
TP112  62.87,85.72 0 top
TP113  69.22,89.53 0 top
TP114  63.5,86.36 0 top
TP115  67.94,81.28 0 top
TP116  67.31,80.64 0 top
TP117  66.67,81.28 0 top
TP118  66.04,80.64 0 top
TP119  71.12,83.19 0 top
TP120  69.22,81.28 0 top
TP121  68.58,80.64 0 top
TP122  62.87,84.45 0 top
TP123  63.5,85.09 0 top
TP124  62.87,83.19 0 top
TP125  65.41,81.28 0 top
TP126  63.5,83.82 0 top
U1  67.31,85.09 270 top
U2  10.16,81.28 180 top
U3  22.86,25.4 0 top
U4  CAT24C32WI-GT3  [SOIC127P600X175-8N']  22.86,32.38 0 top
U$2  57.78,62.87 0 top
U$3  24.13,90.17 0 top

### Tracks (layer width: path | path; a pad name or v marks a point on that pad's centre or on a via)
3V3  (via drill 0.35)
  Top 0.254: TP71.TP 5.11,81.31 6.78,81.31 U2.4 6.93,81.31 13.49,81.31 U2.2 13.56,81.38 14.55,82.37 14.55,84.89 15.16,85.5 | 15.16,85.5 19.2,89.53 20.88,89.53 21.49,88.92 TP59.TP 21.64,88.92 24.08,88.92 U$3.2 24.23,88.92 v27.96,88.92 28.04,89 37.64,89 40.69,92.05 47.55,92.05 v56.01,83.59 | v15.62,85.11 15.54,85.11 15.16,85.5 | U1.6 66.29,87.48 65.84,87.48 U1.7 65.68,87.48 64.01,87.48 63.4,88.09 61.87,88.09 v60.27,86.49 | v48.54,78.18 48.01,77.65 48.01,76.89 R10.1 | U$2.19 U$2.20 62.41,61.04 61.95,61.04 61.19,61.8 | 61.27,69.34 61.19,69.42 61.19,70.26 61.65,70.71 | 61.27,69.34 61.34,69.27 64.47,69.27 66.29,71.09 67.74,71.09 C26.1 | 61.65,70.71 61.95,71.02 62.41,71.02 U$2.28 62.48,71.17 64.08,71.17 TP102.TP 64.24,71.17 66.67,73.61 67.74,73.61 C5.1 67.89,73.76 68.73,74.6 v68.73,75.97 | 61.27,69.34 61.19,69.27 61.19,68.2 62.03,67.36 62.48,67.36 U$2.25 61.95,67.28 61.19,66.52 61.19,61.8 | C4.2 73,60.96 73.61,61.57 J1.4 | v72.01,59.05 71.4,58.45 70.64,58.45 R5.1 | v72.01,56.54 71.32,56.54 70.71,55.93 R6.1 70.56,55.85 69.88,55.85 68.66,54.63 62.56,54.63 U$2.15 62.48,54.56 61.87,53.95 47.93,53.95 47.7,54.18 47.7,54.25 46.41,55.55 R12.1 46.86,55.24 47.85,56.24 49.3,56.24 50.83,57.76 54.1,57.76 58.06,61.72 61.11,61.72 61.19,61.8 | v52.5,79.78 52.58,79.78 61.65,70.71
  Bottom 0.254: R11.2 16.76,85.11 v15.62,85.11 14.71,85.11 12.19,82.6 11.58,82.6 C3.1 | C22.1 29.34,87.02 C21.1 29.26,88.92 v27.96,88.92 | v60.27,86.49 59.51,85.72 R24.1 58.83,85.65 58.22,85.65 56.08,83.52 | v48.54,78.18 50.75,78.18 52.43,79.86 | 56.08,83.52 52.43,79.86 | C20.1 68.73,80.01 68.73,77.5 C19.1 68.73,77.42 v68.73,75.97 | J1.4 73.61,61.57 73.61,61.34 72.01,59.74 v72.01,59.05 v72.01,56.54 | v52.5,79.78 52.43,79.86 | v56.01,83.59 56.08,83.52
BAT  (via drill 0.35)
  Top 0.152: TP82.TP U3.3 20.73,24.77 21.72,23.77 v21.72,21.41
  Bottom 0.152: R19.2 21.72,19.05 v21.72,21.41 21.72,22.86 R20.2
CS_IO18
  Top 0.152: U$2.9 47.62,60.96 45.41,63.18 45.41,76.2 R10.2 46.04,78.42 44.45,80.01 TP29.TP
  Top 0.254: U$3.30 TP29.TP
CTS
  Top 0.152: TP106.TP 70.41,83.82 70.18,84.05 69.72,84.05 U1.23
DCD
  Top 0.152: TP109.TP 69.8,88.85 69.8,88.39 68.89,87.48 U1.1
DSR
  Top 0.152: TP107.TP 71.7,86.33 70.41,86.33 70.18,86.11 69.72,86.11 U1.27
DTR  (via drill 0.35)
  Top 0.152: TP108.TP 46.41,95.94 v46.33,95.94 46.33,93.8 44.96,92.43 21.57,92.43 18.9,89.76 v15.62,89.76 | v44.04,91.06 44.35,91.06 45.72,89.69 45.72,89.08 55.63,79.17 72.24,79.17 75.06,81.99 75.06,85.19 73.3,86.94 71.55,86.94 71.25,86.64 69.72,86.64 U1.28
  Bottom 0.152: Q2.3 46.94,95.02 46.94,95.33 v46.33,95.94 44.04,93.65 v44.04,91.06 | v15.62,89.76 15.62,89.15 15.93,88.85 16.84,88.85 17.14,89.15 17.53,89.15 17.83,88.85 17.91,88.85 18.67,89.61 18.67,90.14 R37.1
EN  (via drill 0.35)
  Top 0.152: 20.57,87.63 20.5,87.63 20.04,88.09 S2.3 20.57,87.63 | 20.57,87.63 TP1.TP U$3.3 | v18.75,95.02 19.96,96.24 19.96,97.23 S2.4 | v20.57,86.56 20.57,87.63
  Bottom 0.152: R11.1 18.75,85.11 18.75,87.25 19.13,87.63 C15.1 19.2,87.63 | 18.63,94.68 18.75,94.79 v18.75,95.02 18.75,96.09 19.13,96.47 C9.1 | 18.63,94.68 18.36,94.41 17.83,94.41 Q1.3 | 19.2,87.63 19.2,88.47 19.96,89.23 19.96,93.34 18.63,94.68 | v20.57,86.56 20.57,86.72 19.66,87.63 19.2,87.63
EXT_5V  (via drill 0.35)
  Top 0.254: MAX232.16 17.83,67.08 15.7,67.08 13.34,64.72 C16.+ | TP83.TP 13.95,85.04 13.95,83.97 13.56,83.59 U2.3 13.41,83.52 6.4,83.52 4.5,81.61 4.5,73 6.33,71.17 SV1.2 | v11.58,66.9 13.79,64.69 C16.+ | U3.8 25.38,27.28 v30.56,27.28 30.63,27.36 58.37,27.36 60.73,29.72 | U4.8 29.64,34.29 v30.48,35.13 30.56,35.2 30.56,53.49 30.63,53.57 30.63,54.18 29.79,55.02 27.2,55.02 26.67,55.55 26.67,57.91 24.16,60.43 | IC1.16 33.6,65.53 33.6,63.86 v33.45,63.7 33.38,63.63 27.36,63.63 24.16,60.43 | 24.16,60.43 21.57,57.84 21.57,52.88 18.44,49.76 C13.- 18.36,49.61 18.36,46.94 SV3.1 14.71,43.13 16.46,41.38 16.46,40.23 15.77,39.55 13.79,39.55 12.34,38.1 SV2.5 6.25,38.18 4.5,39.93 4.5,51.21 5.18,51.89 7.16,51.89 8.15,52.88 8.15,58.83 13.26,63.93 C16.+ | TP87.TP 78.79,81.23 82.6,81.23 POWER.3 83.9,79.93 83.9,78.03 88.85,73.08 88.85,41.6 v86.72,39.47 | PUSH_BUTTON.3 69.19,11.43 71.78,14.02 | 71.78,14.02 74.83,14.02 77.42,11.43 PUSH_BUTTON.7 | 60.73,29.72 60.5,29.95 60.5,33.22 63.7,36.42 RELAY.A1 | 60.73,29.72 71.7,18.75 71.7,14.1 71.78,14.02
  Bottom 0.254: C25.1 19.2,82.53 19.2,80.09 C24.1 19.13,80.01 19.13,79.17 18.29,78.33 15.32,78.33 14.86,78.79 11.58,78.79 C1.1 11.58,78.64 11.58,75.82 7.47,71.7 7.47,71.17 SV1.2 6.4,71.09 7.39,71.09 v11.58,66.9 | R14.1 31.93,19.05 31.93,22.86 R15.1 31.93,22.94 31.93,26.59 R18.2 | R18.2 31.93,26.67 31.93,29.11 R17.1 31.85,29.26 31.85,31.7 C18.1 31.85,31.85 31.85,34.29 C17.1 31.77,34.37 31.24,34.37 v30.48,35.13 | v30.56,27.28 31.85,27.28 R18.2 | R35.1 34.98,63.02 R34.1 34.82,63.02 34.14,63.02 v33.45,63.7 | R35.1 | R36.1 41.22,63.02 38.18,63.02 R35.1 | D1.K 58.29,90.83 59.82,90.83 61.27,92.28 65.08,92.28 65.99,91.36 73.61,91.36 78.56,86.41 79.17,86.41 R2.2 79.25,86.26 79.25,85.57 83.82,81 POWER.3 | 86.72,39.4 81.15,39.4 74.07,32.31 72.47,32.31 71.93,31.77 D3.K 71.78,31.77 71.17,31.77 66.45,36.5 63.78,36.5 RELAY.A1 | 86.72,39.4 87.94,39.4 R22.2 | v86.72,39.47 86.72,39.4
GND  (via drill 0.35)
  Top 0.254: U1.29 67.36,85.11 67.36,86.49 67.74,86.87 67.74,87.4 U1.3 67.82,87.55 67.82,89.15 67.89,89.23 67.89,89.84 67.36,90.37 67.36,90.98 71.02,94.64 72.77,94.64 73,94.87 73,95.17 73.46,95.17 73.53,95.1 73.53,95.04
  Bottom 0.254: C8.2 C7.2
  other vias: 55.88,63.5 43.81,54.61 48.26,71.75 50.8,87 39.37,88.9 64.77,62.87 58.42,57.78 66.04,59.69 22.86,29.84 17.78,33.02 27.3,33.02 41.27,37.47 51.44,95.25 27.3,91.44 21.59,63.5 19.68,60.33 27.94,76.2 16.51,66.04 75.56,71.12 76.83,96.52 71.75,92.71 26.04,37.47 36.2,80.01 34.92,86.36 14.61,74.93 17.78,70.48
  pour Top: 0,100.33 95.25,100.33 95.25,0 0,0
  pour Bottom: 0,100.33 95.25,100.33 95.25,0 0,0
INT_IO23
  Top 0.152: U$2.4 52.07,67.31 50.23,69.15 50.23,80.58 43.81,87 43.81,88.27 TP23.TP 43.13,88.92 41.15,88.92 U$3.37
IO0  (via drill 0.35)
  Top 0.152: U$3.25 41.15,73.69 43.13,73.69 TP34.TP 43.13,73.76 43.13,74.07 43.89,74.83 v43.89,75.74 | v44.73,89.76 44.73,88.16 S1.4 | v45.64,94.03 44.81,94.87 44.81,97.23 S1.3
  Bottom 0.152: 44.81,89.76 44.81,87.86 45.57,87.1 45.57,86.41 C14.1 45.57,86.33 45.57,85.65 43.89,83.97 v43.89,75.74 | 44.81,89.76 44.81,89.84 46.02,91.06 46.02,92.96 Q2.2 45.95,92.96 45.95,93.73 v45.64,94.03 | 44.81,89.76 v44.73,89.76
IO2  (via drill 0.35)
  Top 0.152: U$3.24 38.33,72.69 38.1,72.47 TP22.TP 38.1,71.09 39.62,69.57 v40.39,69.57 | v70.03,31.09 70.03,32.54 49,53.57 46.56,53.57 43.13,57 43.13,66.83 v42.06,67.89 | S3.2 57.15,83.52 v55.4,81.76
  Bottom 0.152: v70.03,31.09 71.86,29.26 71.86,26.06 71.48,25.68 70.18,25.68 70.1,25.76 68.89,25.76 Q4.1 | v40.39,69.57 v42.06,67.89 41.83,68.2 v55.4,81.76
IO4
  Top 0.152: TP33.TP 43.13,74.98 41.15,74.98 U$3.26 41.07,74.91 40.54,74.91 39.85,74.22 39.85,71.48 41.3,70.03 41.3,68.96 40.39,68.05 33.76,68.05 29.72,64.01 26.14,64.01 20.12,57.99 15.62,57.99 8.15,50.52 8.15,50.06 SV2.1
IO12  (via drill 0.35)
  Top 0.152: U$3.14 24.08,73.61 24.08,65.38 23.93,65.23 23.09,65.23 22.94,65.38 22.94,67.51 21.64,68.81 21.64,73.61 TP12.TP 21.03,74.22 21.03,77.72 21.49,78.18 v22.55,78.18 | v37.87,93.04 43.43,98.6 45.72,98.6 54.56,89.76 54.56,88.47 S3.1
  Bottom 0.152: v37.87,93.04 23.01,78.18 v22.55,78.18
IO13  (via drill 0.35)
  Top 0.152: U$3.16 28.12,72.69 27.96,72.54 27.96,71.17 TP14.TP 27.89,71.09 27.89,68.81 26.59,67.51 26.59,65.38 23.24,62.03 12.34,62.03 v10.59,60.27
  Bottom 0.152: v10.59,60.27 7.39,63.48 6.4,63.48 SV1.5
IO15  (via drill 0.35)
  Top 0.152: U$3.23 37.03,72.69 36.88,72.54 36.88,71.17 TP21.TP 36.8,71.09 36.35,71.09 29.57,64.31 25.98,64.31 20.5,58.83 9.6,58.83 v9.37,59.05
  Bottom 0.152: v9.37,59.05 7.47,60.96 SV1.6
IO16  (via drill 0.35)
  Top 0.152: TP32.TP 41.15,76.2 U$3.27 41.07,76.12 39.85,76.12 v38.33,74.6
  Bottom 0.152: v38.33,74.6 6.93,43.2 6.4,43.2 SV2.3
IO32
  Top 0.152: U$3.8 24.08,81.31 21.64,81.31 TP6.TP 21.57,81.23 19.05,81.23 6.4,68.58 SV1.3
IO33
  Top 0.152: U$3.9 TP7.TP 21.57,80.01 21.57,79.48 11.35,69.27 11.35,68.43 8.99,66.06 6.4,66.06 SV1.4
IO34  (via drill 0.35)
  Top 0.152: TP4.TP U$3.6 27.89,83.82 29.03,84.96 34.29,84.96 38.33,80.92 v38.33,75.51 | v39.78,63.86 39.78,61.11 41.99,58.9 41.99,55.17 44.2,52.96 46.1,52.96 57.99,41.07 v57.99,28.04
  Bottom 0.152: R29.1 71.17,6.02 73.15,6.02 73.61,6.48 C23.2 73.69,6.55 74.14,7.01 74.14,13.26 73.08,14.33 71.7,14.33 v57.99,28.04 | v38.33,75.51 39.47,74.37 39.47,64.16 v39.78,63.86
IO35  (via drill 0.35)
  Top 0.152: TP5.TP 21.64,82.6 24.08,82.6 U$3.7 24.16,82.53 25.98,82.53 34.52,73.99 38.94,73.99 39.55,73.38 39.55,71.32 41,69.88 41,69.27 40.39,68.66 v40.08,68.66 | v55.47,53.26 72.54,53.26 83.59,42.22 v87.94,42.22
  Bottom 0.152: Q6.3 87.94,43.13 v87.94,42.22 87.94,41.99 89.84,40.08 89.84,39.4 R22.1 | v55.47,53.26 v40.08,68.66
LEDA
  Top 0.152: U$2.27 62.48,69.88 64.08,69.88 TP66.TP 64.16,69.88 64.54,69.88 66.98,72.31 85.42,72.31 88.47,69.27 88.47,56.62 87.48,55.63 J1.9
LEDB
  Top 0.152: U$2.26 TP65.TP 65.76,68.58 67.13,69.95 77.42,69.95 78.94,71.48 84.81,71.48 87.4,68.89 J1.12
N$1  (via drill 0.35)
  Top 0.152: v82.14,84.89 81.46,85.57 81.46,85.72 LED1.A
  Bottom 0.152: v82.14,84.89 82.14,86.26 82.07,86.33 R2.1
N$2
  Bottom 0.152: Q1.1 18.67,92.28 18.52,92.28 16.84,90.6 16.84,90.22 R37.2
N$3
  Bottom 0.152: Q2.1 47.93,92.96 47.93,91.52 46.02,89.61 46.02,88.92 R21.2
N$4  (via drill 0.35)
  Top 0.152: U1.8 64.92,86.56 64.47,86.56 64.31,86.41 63.55,86.41 TP114.TP 63.48,86.41 63.48,87.02 v63.09,87.4
  Bottom 0.152: R1.1 61.8,88.24 62.26,88.24 v63.09,87.4 63.09,84.05 62.26,83.21 61.8,83.21 R26.2
N$5
  Top 0.152: SV2.4 6.4,40.69 14.55,40.69 SV3.2
N$6  (via drill 0.35)
  Top 0.152: U1.11 64.92,85.11 63.55,85.11 TP123.TP 63.48,85.04 62.64,85.04 62.33,84.73 62.33,81.53 v62.48,81.38
  Bottom 0.152: v62.48,81.38 61.8,80.7 61.34,80.7 R23.1
N$7
  Bottom 0.152: R8.2 83.97,64.16 84.58,64.16 86.72,66.29 87.4,66.29 J1.11
N$8
  Top 0.152: C2.2 70.64,68.58 70.64,66.06 R3.1 70.71,66.06 72.92,66.06 73.91,65.08 74.07,65.08 74.6,64.54 74.6,62.87 | J1.5 TP68.TP 74.6,62.87 | 74.6,62.87 73.61,62.87 73,63.48 70.64,63.48 R4.1
N$9
  Bottom 0.152: R9.2 83.97,60.27 84.96,60.27 87.02,58.22 87.4,58.22 J1.10
N$10
  Top 0.152: TP115.TP 67.89,81.31 67.89,82.6 67.82,82.68 U1.19
N$11
  Top 0.152: TP116.TP 67.36,80.7 67.36,82.68 U1.18
N$12
  Top 0.152: MAX232.1 16.76,56.69 13.34,53.26 C10.+
N$13
  Top 0.152: TP117.TP 66.67,82.6 66.75,82.68 U1.17
N$14
  Top 0.152: MAX232.3 20.95,53.34 18.82,51.21 14.86,51.21 13.34,49.68 C10.-
N$15
  Top 0.152: MAX232.5 23.55,56.69 23.55,53.26 C11.-
N$16  (via drill 0.35)
  Top 0.152: U1.9 64.92,86.03 64.47,86.03 64.16,85.72 TP112.TP 60.5,85.72 v60.35,85.57
  Bottom 0.152: v60.35,85.57 61.57,85.57 61.72,85.72 R24.2
N$17
  Top 0.152: TP118.TP 66.06,80.7 66.06,81.99 66.29,82.22 66.29,82.68 U1.16
N$18
  Top 0.152: MAX232.4 22.25,56.69 22.25,50.9 23.47,49.68 C11.+
N$19
  Top 0.152: MAX232.6 24.77,56.24 27.74,53.26 28.57,53.26 C12.-
N$20
  Top 0.152: MAX232.2 19.66,56.69 19.66,54.48 18.44,53.26 C13.+
N$21
  Top 0.152: RELAY_CONN.5 81.69,36.42 75.97,36.42 RELAY.NC
N$22
  Top 0.152: RELAY.COM 82.6,30.48 83.82,29.26 RELAY_CONN.3
N$23
  Top 0.152: LED2.C 33.68,49.99 35.05,49.99 35.51,49.53 LED5.K
  Bottom 0.152: LED5.K 34.82,49.53 34.37,49.99 33.68,49.99 R31.1
N$24
  Top 0.152: R40NC.2 30.48,62.1 34.52,62.1 37.41,65 37.41,65.53 IC1.13
N$25
  Top 0.152: TP119.TP 71.09,83.21 70.03,83.21 69.72,83.52 U1.22
N$26
  Top 0.152: RELAY.NO 75.97,24.46 83.52,24.46 83.82,24.16 RELAY_CONN.1
N$27
  Bottom 0.152: 69.23,29.76 67.82,31.17 67.82,31.7 D3.A | 69.23,29.76 70.87,28.12 70.87,26.67 Q4.3 | 69.23,29.76 64.01,24.54 63.78,24.54 RELAY.A2
N$28  (via drill 0.35)
  Top 0.152: v22.55,32.31 19.36,32.31 17.45,30.4 15.93,30.4 D2.A
  Bottom 0.152: v22.55,32.31 23.39,32.31 23.47,32.38 25.38,32.38 28.5,29.26 29.03,29.26 R17.2
N$29  (via drill 0.35)
  Top 0.152: D2.K 15.85,34.37 14.02,32.54 14.02,29.26 TP78.TP 14.02,29.18 14.48,28.73 v16.08,28.73 | v32.46,35.74 33.98,35.74 37.95,31.77 56.31,31.77 BT1.+
  Bottom 0.152: R20.1 18.9,25.91 17.03,27.77 | v16.08,28.73 17.03,27.77 | R20.1 | v32.46,35.74 32.31,35.89 25.15,35.89 17.03,27.77
N$30
  Top 0.152: TP120.TP 69.19,81.31 69.19,82.37 68.89,82.68 U1.21
N$31
  Top 0.152: TP121.TP 68.58,81.99 68.35,82.22 68.35,82.68 U1.20
N$32
  Bottom 0.152: R27.1 89.46,45.72 89.46,44.88 89.84,44.5 89.84,44.2 Q6.1
N$33
  Bottom 0.152: 69.8,4.12 71.09,4.12 R29.2 | 69.8,4.12 67.36,4.12 R28.2 | 69.8,4.12 69.8,7.09 72.39,9.68 PUSH_BUTTON.5
N$34
  Top 0.152: TP122.TP 62.87,84.51 64.85,84.51 64.92,84.58 U1.12
N$35
  Bottom 0.152: R27.2 87.86,45.72 83.82,49.76 DRY_CONTACT.3
N$36
  Top 0.152: LED2.A 33.68,51.59 35.05,51.59 35.51,52.05 LED5.A 35.59,52.12 37.41,53.95 37.41,56.31 IC1.4
N$37
  Top 0.152: LED6.A 40.16,51.59 38.79,51.59 LED3.A 38.79,51.66 38.79,56.31 IC1.5
N$38
  Top 0.152: 43.81,51.59 45.26,51.59 45.72,52.05 LED7.A | IC1.6 40.01,55.4 43.81,51.59 | 43.81,51.59 LED4.A
N$39
  Top 0.152: TP124.TP 62.87,83.21 64.62,83.21 64.92,83.52 U1.14
N$40
  Bottom 0.152: R30.2 64.77,4.19 63.93,5.03 63.55,5.03 62.94,5.64 62.94,8.91 62.26,9.6 62.26,11.43 PUSH_BUTTON.1
N$41
  Top 0.152: TP125.TP 65.46,81.31 65.46,82.37 65.76,82.68 U1.15
N$42
  Top 0.152: TP126.TP 64.24,83.82 64.47,84.05 64.92,84.05 U1.13
N$45  (via drill 0.35)
  Top 0.152: TP89.TP 33.68,54.63 33.68,56.31 IC1.1 33.6,56.39 31.97,58.03 | R40NC.1 30.48,59.51 31.97,58.03 | 31.97,58.03 v33.45,59.51
  Bottom 0.152: v33.45,59.51 34.06,60.12 34.9,60.12 R34.2
N$46  (via drill 0.35)
  Top 0.152: TP90.TP 34.98,54.63 34.98,56.31 IC1.2 34.98,56.39 34.98,56.92 36.88,58.83 v37.26,58.83
  Bottom 0.152: R35.2 38.1,59.66 v37.26,58.83
N$47  (via drill 0.35)
  Top 0.152: TP91.TP IC1.3 36.2,56.84 39.55,60.2 v39.78,60.2
  Bottom 0.152: v39.78,60.2 41.22,60.2 R36.2
N$48
  Top 0.152: LED3.C 38.79,49.99 40.16,49.99 40.62,49.53 LED6.K
  Bottom 0.152: LED6.K 39.85,49.53 39.4,49.99 38.79,49.99 R32.1
N$49
  Top 0.152: LED7.K 45.26,49.99 43.81,49.99 LED4.C
  Bottom 0.152: LED7.K 44.96,49.53 44.5,49.99 43.81,49.99 R33.1
N$67
  Top 0.152: TP20.TP 35.59,71.17 35.59,72.54 35.74,72.69 U$3.22
N$68
  Top 0.152: TP19.TP 34.29,72.47 34.52,72.69 U$3.21
N$69
  Top 0.152: TP18.TP 33.07,71.17 33.07,72.54 33.22,72.69 U$3.20
N$70
  Top 0.152: TP17.TP 31.77,71.17 31.77,72.54 31.93,72.69 U$3.19
N$71
  Top 0.152: TP16.TP 30.48,72.47 30.71,72.69 U$3.18
N$72
  Top 0.152: TP15.TP 29.26,71.17 29.26,72.54 29.41,72.69 U$3.17
OS1
  Top 0.152: U3.1 20.34,27.36 18.44,27.36 TP80.TP 18.36,27.36 15.93,27.36 Q5.1
OS2
  Top 0.152: U3.2 20.34,26.06 18.44,26.06 TP85.TP 18.36,25.98 15.93,25.98 Q5.2
OSC1  (via drill 0.35)
  Top 0.152: U$2.23 63.63,64.77 64.62,65.76 64.62,66.37 v64.01,66.98
  Bottom 0.152: v64.01,66.98 62.87,68.12 61.04,68.12 60.43,68.73 C7.1 60.35,68.73 60.35,70.94 60.43,71.02 60.43,71.4 60.35,71.48 60.35,71.7 TP54.TP 60.27,71.78 60.27,72.01 59.66,72.62 59.66,73.46 60.27,74.07 60.27,74.91 Q3.2
OSC2  (via drill 0.35)
  Top 0.152: v64.01,66.06 62.48,66.06 U$2.24
  Bottom 0.152: v64.01,66.06 62.71,67.36 57.3,67.36 56.01,68.66 55.24,68.66 C8.1 55.24,68.73 54.71,69.27 54.71,71.09 55.24,71.63 TP64.TP 55.24,72.01 54.94,72.31 54.94,73.38 55.24,73.69 Q3.1
RBIAS
  Top 0.152: 51.44,54.63 53.03,54.63 U$2.14 | 51.44,54.63 50.98,55.09 48.92,55.09 R13.2 | 51.44,54.63 TP53.TP
RESET
  Top 0.152: U$2.10 53.03,59.74 51.44,59.74 TP55.TP 51.44,59.66 48.54,59.66 46.41,57.53 R12.2
RI
  Top 0.152: TP113.TP 69.19,89.53 69.19,88.77 68.35,87.94 68.35,87.48 U1.2
RTS  (via drill 0.35)
  Top 0.152: U1.24 69.72,84.58 69.8,84.51 71.09,84.51 TP105.TP 71.17,84.43 71.93,84.43 72.31,84.05 72.31,83.59 68.81,80.09 62.87,80.09 57.99,84.96 57.99,90.6 49.99,98.6 48.39,98.6 47.51,97.73 | v17.14,93.34 37.26,93.34 42.82,98.91 46.33,98.91 47.51,97.73 | v48.01,97.23 47.51,97.73
  Bottom 0.152: v17.14,93.34 16.84,93.04 16.84,92.35 Q1.2 | v48.01,97.23 48.01,94.56 48.92,93.65 48.92,90.6 47.93,89.61 47.93,88.92 R21.1
RX_232
  Top 0.152: MAX232.7 25.98,56.69 25.98,57.15 25.15,57.99 24.38,57.99 24.16,57.76 24.16,55.02 24.54,54.63 24.54,45.19 8.15,28.8 8.15,24.61 6.4,22.86 RS232.3 6.33,22.86 4.57,21.11 4.57,13.87 9.53,8.91 10.74,8.91 13.26,11.43 J2.3
RX_S  (via drill 0.35)
  Top 0.152: MAX232.14 20.95,66.06 19.51,64.62 v14.86,64.62 | v10.74,68.73 8.69,68.73 7.01,67.06 5.18,67.06 3.81,65.68 3.81,13.72 9.22,8.31 48.92,8.31 52.05,11.43 SCANNER.7
  Bottom 0.152: v10.74,68.73 v14.86,64.62
RX_UART1_IO14
  Top 0.152: 22.86,74.98 24.08,74.98 U$3.13 | 22.86,74.98 21.64,74.98 TP11.TP | 22.86,74.98 22.86,73.15 23.47,72.54 23.47,66.52 MAX232.12
RX_UART2_IO25
  Top 0.152: TP8.TP 21.64,78.79 24.08,78.79 U$3.10
RXD
  Top 0.152: U1.25 69.72,85.11 71.7,85.11 TP103.TP 71.78,85.04 72.62,84.2 72.62,84.12 74.14,82.6 R39.2
RXD0  (via drill 0.35)
  Top 0.152: U$3.34 41.15,85.11 43.13,85.11 TP26.TP 43.2,85.04 45.95,82.3 v47.02,82.3 | v50.44,85.72 56.39,79.78 68.96,79.78 71.7,82.53 73.15,82.53 R39.1
  Bottom 0.152: v47.02,82.3 v50.44,85.72
SCK_IO19
  Top 0.152: U$3.31 TP28.TP 44.45,81.28 46.92,78.81 46.92,75.99 45.72,74.79 45.72,63.5 46.99,62.23 U$2.8
SCL_IO5  (via drill 0.35)
  Top 0.152: U3.6 27.36,24.77 | 27.36,24.77 TP30.TP | v27.81,27.96 27.89,28.04 27.89,30.71 27.36,31.24 27.36,31.7 TP79.TP 27.36,31.77 28.5,31.77 31.85,35.13 31.85,52.05 34.37,54.56 34.37,60.73 38.02,64.39 38.02,67.44 | v23.77,31.77 25.3,31.77 U4.6 | v27.36,25.38 27.36,24.77 | U$3.29 41.15,78.79 43.13,78.79 TP86.TP 44.81,77.11 44.81,71.55 40.69,67.44 38.02,67.44 | IC1.14 36.2,66.06 37.57,67.44 38.02,67.44
  Bottom 0.152: 27.66,25.38 27.66,24.99 29.03,23.62 29.03,22.86 R15.2 | 27.66,25.38 27.66,27.81 v27.81,27.96 27.66,27.89 v23.77,31.77 | 27.66,25.38 v27.36,25.38
SDA_IO17  (via drill 0.35)
  Top 0.152: 25.26,28.23 24.92,27.89 24.31,27.89 24.08,27.66 24.08,24.46 24.99,23.55 25.3,23.55 U3.5 25.38,23.55 27.89,23.55 TP31.TP 29.03,22.4 v29.03,20.5 | 25.26,28.23 27.28,30.25 27.28,30.48 TP81.TP | 25.3,30.48 25.3,29.64 v25.15,29.49 | v25.15,28.27 25.22,28.27 25.26,28.23 | U$3.28 41.15,77.5 43.13,77.5 TP88.TP 43.2,77.42 44.5,76.12 44.5,71.7 40.54,67.74 36.65,67.74 34.98,66.06 34.98,65.61 IC1.15 34.9,65.53 34.9,64.24 33.76,63.09 30.48,63.09 29.87,62.48 29.87,60.66 29.95,60.58 v29.95,56.01 | 25.3,30.48 24.16,30.48 23.16,31.47 23.16,41.76 29.95,48.54 v29.95,53.87 | 25.3,30.48 U4.5
  Bottom 0.152: v29.03,20.5 29.03,19.05 R14.2 | v25.15,28.27 v25.15,29.49 | v29.95,56.01 v29.95,53.87
SENSOR_VN
  Top 0.152: TP3.TP 21.64,85.11 24.08,85.11 U$3.5
SENSOR_VP
  Top 0.152: TP2.TP 21.64,86.33 24.08,86.33 U$3.4
SI_IO21
  Top 0.152: U$2.7 50.8,63.5 50.16,62.87 46.99,62.87 46.02,63.83 46.02,72.69 49.53,76.2 49.53,78.11 43.81,83.82 TP27.TP U$3.33
SO_IO22
  Top 0.152: U$2.6 52.76,64.77 49.92,67.61 49.92,80.36 43.18,87.11 TP24.TP U$3.36
SQ  (via drill 0.35)
  Top 0.152: U3.7 25.38,26.06 27.89,26.06 TP84.TP 27.96,25.98 v28.73,25.22
  Bottom 0.152: v28.73,25.22 29.03,25.53 29.03,26.67 R18.1
TPIN+
  Top 0.152: J1.3 76.2,60.36 74.04,62.52 73.28,62.52 72.99,62.23 69.06,62.23 R4.2 65.41,61.11 65.41,59.69 63.5,57.78 60.96,57.78 59.05,55.88 U$2.13 TP57.TP
TPIN-
  Top 0.152: TP56.TP U$2.12 54.04,57.15 55.95,59.05 63.44,59.05 64.34,59.95 64.34,60.53 66.76,62.95 66.76,64.5 67.79,65.53 R3.2 69.2,64.63 71.53,64.63 72.03,64.13 J1.6
TPOUT+
  Top 0.152: U$2.17 TP63.TP 65.41,58.42 R5.2 69.06,59.69 72.39,59.69 73.03,60.33 74.3,60.33 76.2,58.42 J1.1
TPOUT-
  Top 0.152: U$2.16 TP62.TP R6.2 69.06,57.15 72.39,57.15 73.66,58.42 J1.2
TX_232
  Top 0.152: MAX232.8 28.35,56.69 29.64,55.4 29.95,55.4 31.09,54.25 31.09,34.82 28.57,32.31 27.05,32.31 26.59,31.85 26.59,30.02 25.45,28.88 17.14,28.88 16.38,28.12 14.17,28.12 6.4,20.34 RS232.4 10.13,16.54 10.13,11.43 J2.1
TX_S
  Top 0.152: MAX232.13 22.17,66.52 22.17,66.98 21.41,67.74 11.51,67.74 8.15,64.39 8.15,60.58 7.01,59.44 5.18,59.44 4.12,58.37 4.12,13.87 9.37,8.61 44.12,8.61 46.94,11.43 SCANNER.5
TX_UART1_IO27
  Top 0.152: TP10.TP U$3.12 24.69,76.2 25.38,75.51 25.38,73.08 24.77,72.47 MAX232.11
TX_UART2_IO26
  Top 0.152: TP9.TP 21.64,77.5 24.08,77.5 U$3.11 24.16,77.42 24.69,77.42 25.98,76.12 25.98,66.52 MAX232.10
TXD
  Top 0.152: U1.26 69.72,85.65 69.8,85.72 TP104.TP 73.53,85.72 74.14,85.11 R38.2
TXD0
  Top 0.152: TP25.TP 43.13,86.41 41.15,86.41 U$3.35 41.07,86.41 40.54,86.41 38.58,88.37 38.58,89.41 40.84,91.67 44.35,91.67 46.02,89.99 46.02,89.23 55.78,79.48 72.08,79.48 74.75,82.14 74.75,82.98 73.23,84.51 73.23,85.04 R38.1
USB_DN
  Top 0.152: TP111.TP 77.5,90.83 77.5,92.2 J4.2 77.5,92.28 77.5,92.81 78.41,93.73 78.94,93.73 79.17,93.95 79.17,96.01 77.62,97.56 67.77,97.56 65.95,95.75 | U1.5 66.75,87.48 66.67,87.55 TP99.TP 66.67,88.92 64.92,88.92 62.48,91.36 62.48,95.78 63.32,96.62 65.08,96.62 65.95,95.75 | 65.95,95.75 65.99,95.71 65.99,95.02 J3.2
USB_DP  (via drill 0.35)
  Top 0.152: U1.4 67.36,87.48 67.36,89.53 TP100.TP 67.28,89.53 v66.67,90.14 | TP110.TP 76.2,90.98 76.81,91.59 76.81,92.2 J4.3 76.81,92.28 76.81,92.81 76.43,93.19 75.21,93.19 74.56,93.84 | J3.3 66.67,95.71 67.59,96.62 73.91,96.62 74.52,96.01 74.52,93.88 74.56,93.84 | v68.05,90.68 71.4,90.68 74.56,93.84
  Bottom 0.152: v66.67,90.14 67.51,90.14 v68.05,90.68
VBUS  (via drill 0.35)
  Top 0.254: v70.03,89.76 70.26,89.53 77.04,89.53 78.11,90.6 78.11,92.2 J4.1 | v65.23,89.53 65.23,93.42 65.3,93.5 65.3,94.94 J3.1
  Bottom 0.254: v70.03,89.76 69.72,89.46 65.23,89.46 | 65.23,89.46 64.47,89.46 63.17,90.75 62.41,90.75 D1.A 62.26,90.83 61.65,90.83 60.35,89.53 60.35,89.15 59.51,88.32 58.98,88.32 R1.2 | v65.23,89.53 65.23,89.46
VCAP
  Top 0.152: TP50.TP 51.44,71.17 53.03,71.17 U$2.1 53.11,71.09 53.49,71.09 54.33,70.26 54.33,64.39 54.18,64.24 51.97,64.24 48.92,67.28 48.92,68.43 C6.+

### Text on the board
tNames: +5V | GND | LCD | SIG | GND | ParkMe | TX | RX | NC | GND | GND | NC | TX | -VE | +VE | PB | PB | PRINTER | RX
bNames: NC | COM | NO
